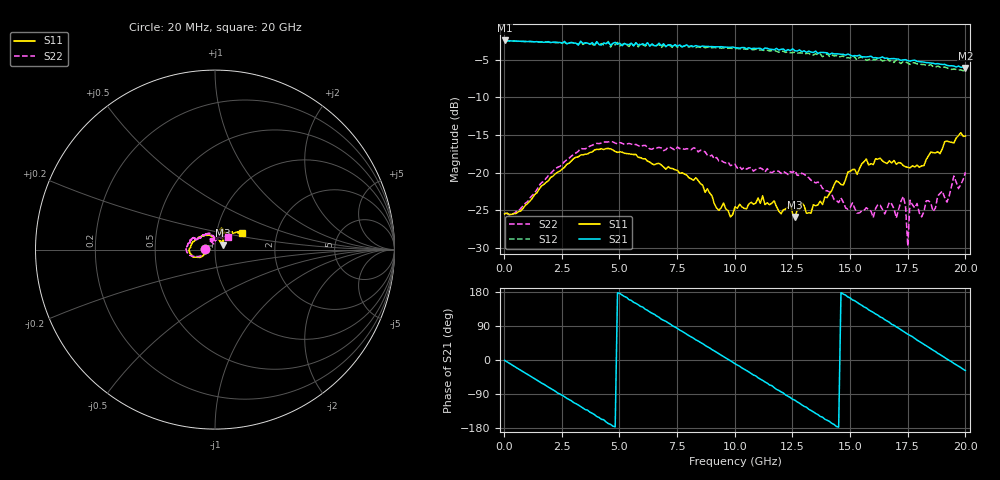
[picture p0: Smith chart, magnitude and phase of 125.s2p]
!Agilent Technologies,N5230A,US43500223,A.07.50.48
!Agilent N5230A: A.07.50.48
!Date: Wednesday, October 07, 2015 19:47:25
!Correction: S11(Full 2 Port(1,2))
!S21(Full 2 Port(1,2))
!S12(Full 2 Port(1,2))
!S22(Full 2 Port(1,2))
!S2P File: Measurements: S11, S21, S12, S22:
# Hz S  RI  R 50
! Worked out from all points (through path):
!   201 points, 20 MHz to 20 GHz, reference 50 ohm
!   highest |S21| = -2.40 dB at 20 MHz (marker M1); lowest = -6.1 dB at 20 GHz (marker M2)
!   group delay of S21, straight-line fit = 104 ps
!   lowest |S11| = -25.9 dB at 12.61 GHz (marker M3), VSWR 1.11, Z = 54.7 + j2.51 ohm
!   |S11| at or under -10 dB: start of sweep to end of sweep
!   |S22| runs from -29.8 to -15.9 dB; largest |S21 - S12| = 0.049
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2e7  -0.0531 0.000909  0.7583 -0.0111  0.7573 -0.0119  -0.0537 0.00139
1.8182e9  -0.0757 -0.0407  0.2797 -0.6858  0.2701 -0.6879  -0.0843 -0.0358
2.6174e9  -0.0997 -0.0424  -0.0883 -0.7421  -0.0922 -0.7302  -0.1114 -0.0398
3.4166e9  -0.1259 -0.0364  -0.4321 -0.5795  -0.4442 -0.559  -0.1406 -0.03
4.9151e9  -0.1355 0.0139  -0.7138 0.034  -0.7341 0.057  -0.1544 0.0158
5.7143e9  -0.1254 0.0409  -0.6295 0.3717  -0.6228 0.3842  -0.1501 0.0348
6.7133e9  -0.0935 0.0672  -0.2824 0.6695  -0.2615 0.6672  -0.1393 0.0471
8.1119e9  -0.0431 0.0797  0.3397 0.6113  0.3511 0.597  -0.1301 0.0569
9.1109e9  -0.00223 0.0621  0.6281 0.2815  0.6297 0.2607  -0.1088 0.0579
1.001e10  0.0371 0.0461  0.6691 -0.1144  0.6566 -0.1296  -0.095 0.0624
1.13087e10  0.0492 0.0362  0.3586 -0.5722  0.3202 -0.5608  -0.0611 0.0802
1.26074e10  0.0451 0.0229  -0.1797 -0.6227  -0.2058 -0.5983  -0.0459 0.0924
1.34066e10  0.0449 0.0412  -0.4596 -0.4314  -0.4464 -0.4103  -0.0199 0.0847
1.51049e10  0.0476 0.0933  -0.555 0.219  -0.5546 0.2352  -0.00585 0.0625
1.67033e10  0.0291 0.1161  -0.0955 0.564  -0.0639 0.5492  -0.0225 0.0594
1.7003e10  0.0286 0.1099  0.0262 0.5705  0.0507 0.5615  -0.00848 0.0491
1.73027e10  0.0374 0.1051  0.1375 0.5462  0.1455 0.5292  -0.00991 0.0686
1.75025e10  0.0357 0.1024  0.21 0.5153  0.2297 0.4844  -0.00675 0.0316
1.76024e10  0.0395 0.1  0.2358 0.4995  0.2352 0.4696  -0.0347 0.0555
1.81019e10  0.0556 0.0957  0.3853 0.3874  0.3794 0.3621  0.0011 0.0507
1.88012e10  0.0953 0.0995  0.5069 0.1613  0.4921 0.1421  0.0164 0.0679
2e10  0.1499 0.0898  0.4389 -0.2331  0.4113 -0.2478  0.0698 0.0721
